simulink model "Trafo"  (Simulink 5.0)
settings: Solver=ode45  StartTime=0.0  StopTime=10.0  MaxStep=0.5e-3  RelTol=1e-6

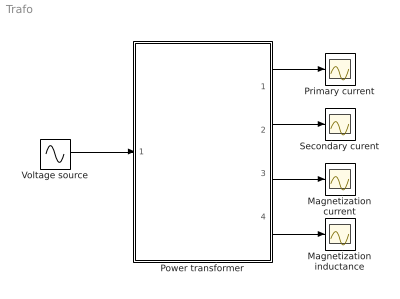
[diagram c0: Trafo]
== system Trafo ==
  Magnetization current : Scope
  Magnetization inductance : Scope
  Power transformer : Subsystem  mask{Sni=1, Vn=400, fn=50, Vscp=6, Pscp=3, I10p=4, Bc0=1.5, Rs=160, fname='MagTrafo1.mat'}
      mask prompts: Sni "Sn (kW)"; Vn "Vn (V)"; fn "fn (Hz)"; Vscp "Vsc (%)"; Pscp "Psc (%)"; I10p "I10 (%)"; Bc0 "Bc0 (T)"; Rs "Rs (Ohm)"; fname "Magnetization curve file"
      mask init:
      | load(fname);
      | Sn=Sni*1000;
      | In=Sn/Vn*sqrt(1+2*Pscp/100+(Vscp/100)^2+(I10p/100)^2);
      | Ib=interp1(Bc,I01ref,Bc0);
      | Lb=interp1(Bc,Lmref,Bc0);
      | I10n=In*I10p/100;
      | Lmn=Vn/(2*pi*fn*I10n);
      | Imref=I01ref*I10n*sqrt(2)/Ib;
      | Lmref2=Lmref*Lmn/Lb;
      | Rsc=Pscp*Sn/(100*In^2)
      | R1=0.5*Rsc;
      | R2=Rsc-R1;
      | Xsc=sqrt((Vscp*Vn/(100*In))^2-Rsc^2);
      | Lsc=Xsc/(2*pi*fn);
      | L1sig=0.5*Lsc;
      | L2sig=Lsc-L1sig;
      | dLmdi=diff(Lmref2)./diff(Imref);
      | Lmtrref=Lmref2(2:end-1)+0.5*(dLmdi(1:end-1)+dLmdi(2:end)).*Imref(2:end-1);
      | Lmtrref=[Lmtrref(1) Lmtrref];
      | Imref=Imref(1:end-1);
      | I0max=Imref(end);
      | I0=(I0max*Lmtrref(end)-Imref(end-1)*Lmtrref(end-1))/(Lmtrref(end-1)-I0max);
      | kl=(I0max+I0)*Lmtrref(end);
  Primary current : Scope
  Secondary curent : Scope
  Voltage source : Sin  Amplitude=400*sqrt(2)  Frequency=100*pi  SampleTime=0
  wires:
  Voltage source/1 -> Power transformer/1("V1 ")
  Power transformer/1(i1) -> Primary current/1
  Power transformer/2(i2) -> Secondary curent/1
  Power transformer/3(i0) -> Magnetization current/1
  Power transformer/4(i3) -> Magnetization inductance/1

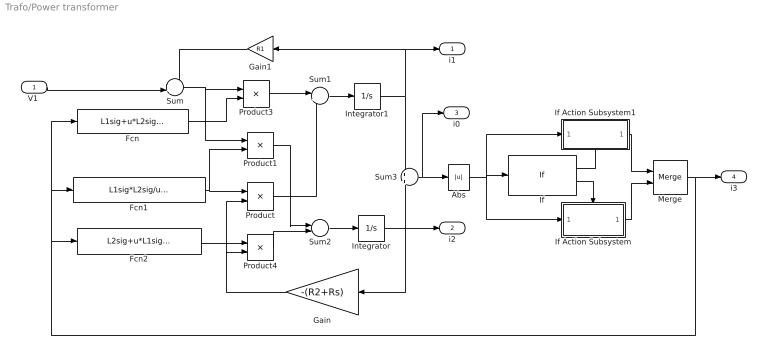
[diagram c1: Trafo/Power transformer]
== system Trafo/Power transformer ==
  "V1 " : Inport
  Abs : Abs
  Fcn : Fcn  Expr=L1sig+u*L2sig/(u+L2sig)
  Fcn1 : Fcn  Expr=L1sig*L2sig/u+L1sig+L2sig
  Fcn2 : Fcn  Expr=L2sig+u*L1sig/(u+L1sig)
  Gain : Gain  Orientation=left  Gain=-(R2+Rs)
  Gain1 : Gain  Orientation=left  Gain=R1
  If : If  IfExpression=u1 < I0max
  If Action Subsystem : Subsystem  TreatAsAtomicUnit=on
  If Action Subsystem1 : Subsystem  TreatAsAtomicUnit=on
  Integrator : Integrator
  Integrator1 : Integrator
  Merge : Merge
  Product : Product  Inputs=/*
  Product1 : Product  Inputs=*/
  Product3 : Product  Inputs=*/
  Product4 : Product  Inputs=/*
  Sum : Sum  Inputs=-+|
  Sum1 : Sum  Inputs=|+-
  Sum2 : Sum  Inputs=|-+
  Sum3 : Sum  Inputs=+|+
  i1 : Outport
  i2 : Outport  Port=2
  i0 : Outport  Port=3
  i3 : Outport  Port=4
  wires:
  Product3/1 -> Sum1/1
  Sum1/1 -> Integrator1/1
  Sum2/1 -> Integrator/1
  Product/1 -> Sum1/2
  Product1/1 -> Sum2/1
  Product4/1 -> Sum2/2
  Gain/1 -> Product/2, Product4/2
  "V1 "/1 -> Sum/2
  Gain1/1 -> Sum/1
  Sum/1 -> Product3/1, Product1/1
  Fcn1/1 -> Product/1, Product1/2
  Fcn/1 -> Product3/2
  Fcn2/1 -> Product4/1
  Integrator/1 -> Gain/1, Sum3/2, i2/1
  Abs/1 -> If/1, If Action Subsystem/1(In1), If Action Subsystem1/1(In1)
  If/2 -> If Action Subsystem/Action
  If/1 -> If Action Subsystem1/Action
  If Action Subsystem1/1(Out1) -> Merge/1
  If Action Subsystem/1(Out1) -> Merge/2
  Merge/1 -> Fcn/1, Fcn1/1, Fcn2/1, i3/1
  Integrator1/1 -> Sum3/1, Gain1/1, i1/1
  Sum3/1 -> Abs/1, i0/1

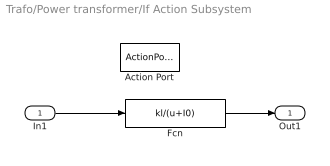
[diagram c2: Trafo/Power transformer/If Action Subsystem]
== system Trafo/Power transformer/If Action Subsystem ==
  In1 : Inport
  Action Port : ActionPort  ActionType=else
  Fcn : Fcn  Expr=kl/(u+I0)
  Out1 : Outport
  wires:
  In1/1 -> Fcn/1
  Fcn/1 -> Out1/1

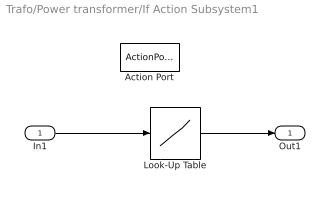
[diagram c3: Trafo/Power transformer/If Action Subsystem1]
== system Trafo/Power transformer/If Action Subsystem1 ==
  In1 : Inport
  Action Port : ActionPort  ActionType=then
  Look-Up Table : Lookup  InputValues=Imref  OutputValues=Lmtrref
  Out1 : Outport
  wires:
  In1/1 -> Look-Up Table/1
  Look-Up Table/1 -> Out1/1
